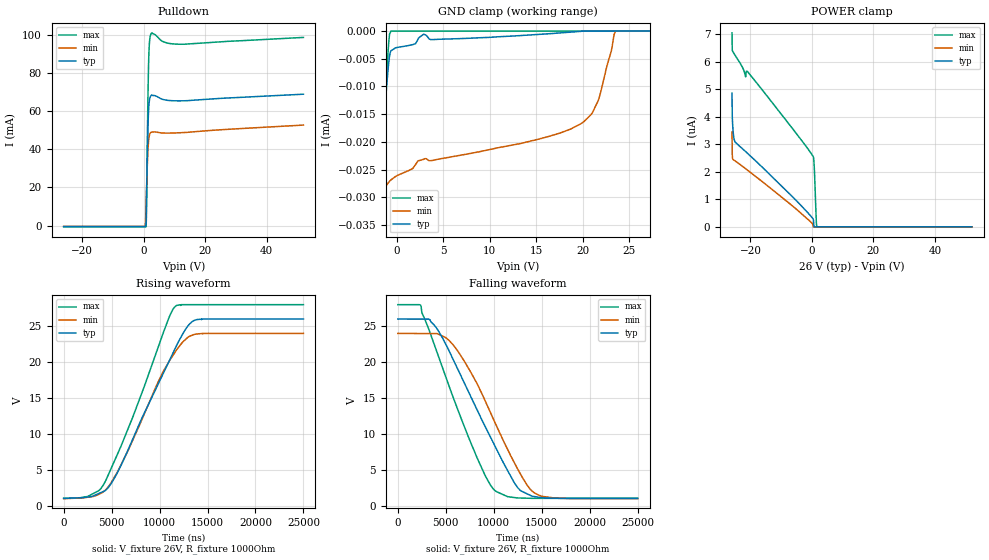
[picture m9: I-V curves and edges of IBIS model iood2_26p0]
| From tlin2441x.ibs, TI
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|   iood2_26p0 Model
[Model]   iood2_26p0
Model_type   I/O_open_drain
Polarity   Non-Inverting
Enable   Active-Low
Vinl = 5.2
Vinh = 22.1
Vmeas = 13
Vref = 26
Cref = 2pF
Rref = 1000
|   typ   min   max
C_comp   6.104pF   6.021pF   6.541pF
|  Where Nom  PVT is Nominal Process, 26.0V,   27C
|   Fast PVT is Strong Process,  28.0,   -40C
|   Slow PVT is Weak Process,   24.0V,   150C
[Model spec]
|subparameter
Vinl   5.2   4.8   5.6
Vinh   22.1   20.4   23.8
[Voltage Range]   26   24   28
|Junction Temperature
[Temperature Range]   27   150   -40
[Pullup Reference]   26   24   28
[Pulldown Reference]   0   0   0
[Power Clamp Reference]   26   24   28
[GND Clamp Reference]   0   0   0
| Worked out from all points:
|   slope of the pulldown table from 0 to 3.9 V, typ, clamps not added: 56.8 ohm
|   falling waveform, V_fixture 26V, R_fixture 1000Ohm: 20-80 % time 5.45us typ, 5.05us min, 4.59us max; typ from 26 V to 1.06 V
|   rising waveform, V_fixture 26V, R_fixture 1000Ohm: 20-80 % time 5.19us typ, 4.75us min, 4.64us max; typ from 1.06 V to 26 V
[Pulldown]
|   Voltage   I(typ)   I(min)   I(max)
-26V      -559.3uA   -442uA     -700.8uA
286mV     -542.5uA   -413.3uA   -677.1uA
598mV     -529.8uA   1.184mA    -668.8uA
754mV     366.6uA    8.145mA    -648.8uA
832mV     4.307mA    12.52mA    -217.7uA
910mV     10.89mA    16.89mA    4.302mA
1.378V    49.24mA    38.19mA    63.69mA
1.69V     62.48mA    45.49mA    88.85mA
2.002V    66.71mA    48.03mA    97.9mA
2.626V    68.6mA     49.05mA    101.2mA
11.13V    65.52mA    48.71mA    95.31mA
52V       69.02mA    52.79mA    98.87mA
[GND Clamp]
|   Voltage   I(typ)   I(min)   I(max)
-26V      -566.7uA   -506.9uA   -646.9uA
-2.288V   -35.25uA   -36.59uA   -36.47uA
-1.82V    -24.99uA   -30.95uA   -24.67uA
-962mV    -6.981uA   -27.44uA   -3.676uA
-806mV    -4.513uA   -27.13uA   -554.1nA
-650mV    -3.578uA   -26.87uA   0A
2.86V     -573.3nA   -23.17uA   0A
13.47V    -797.4nA   -20.24uA   0A
19.94V    -37.25nA   -16.58uA   0A
21.66V    0A         -12.61uA   0A
23.53V    0A         0A         0A
52V       0A         0A         0A
[POWER Clamp]
|   Voltage   I(typ)   I(min)   I(max)
-26V      4.861uA    3.452uA    7.055uA
-25.92V   4.035uA    2.626uA    6.418uA
-25.84V   3.837uA    2.498uA    6.395uA
-25.45V   3.274uA    2.432uA    6.319uA
-24.99V   3.085uA    2.398uA    6.235uA
-21.55V   2.735uA    2.112uA    5.456uA
-20.93V   2.672uA    2.059uA    5.641uA
442mV     276nA      0A         2.551uA
754mV     0A         0A         2.172uA
1.456V    0A         0A         107.9nA
1.612V    0A         0A         0A
52V       0A         0A         0A
[Ramp]
R_load = 1000
|   typ   min   max
dV/dt_r   14.9599/5.17419e-06   13.7828/4.72865e-06   16.1514/4.63927e-06
dV/dt_f   14.9599/5.44556e-06   13.7828/5.04377e-06   16.1514/4.58508e-06
[Falling Waveform]
V_fixture = 26V
V_fixture_min = 24V
V_fixture_max = 28V
R_fixture = 1000Ohm
C_fixture = 0F
|   Time   V(typ)   V(min)   V(max)
0s        26V        24V        28V
2.379us   25.99V     23.99V     27.92V
3.343us   25.9V      23.98V     24.15V
5.675us   20.64V     22.55V     15.45V
8.31us    13.25V     16.88V     6.562V
10.12us   8.382V     11.64V     2.165V
12.5us    2.552V     5.134V     1.128V
14.2us    1.327V     1.864V     1.077V
16.44us   1.092V     1.111V     1.077V
25us      1.065V     1.028V     1.078V
[Rising Waveform]
V_fixture = 26V
V_fixture_min = 24V
V_fixture_max = 28V
R_fixture = 1000Ohm
C_fixture = 0F
|   Time   V(typ)   V(min)   V(max)
0s        1.065V     1.028V     1.078V
2.504us   1.256V     1.228V     1.337V
4.132us   2.028V     1.979V     2.923V
5.509us   4.416V     4.519V     6.918V
7.238us   9.415V     9.27V      12.48V
10.99us   20.15V     20.1V      26.25V
11.69us   22.09V     21.54V     27.81V
12.8us    24.76V     23.27V     28V
13.87us   25.92V     23.92V     28V
25us      26V        24V        28V
